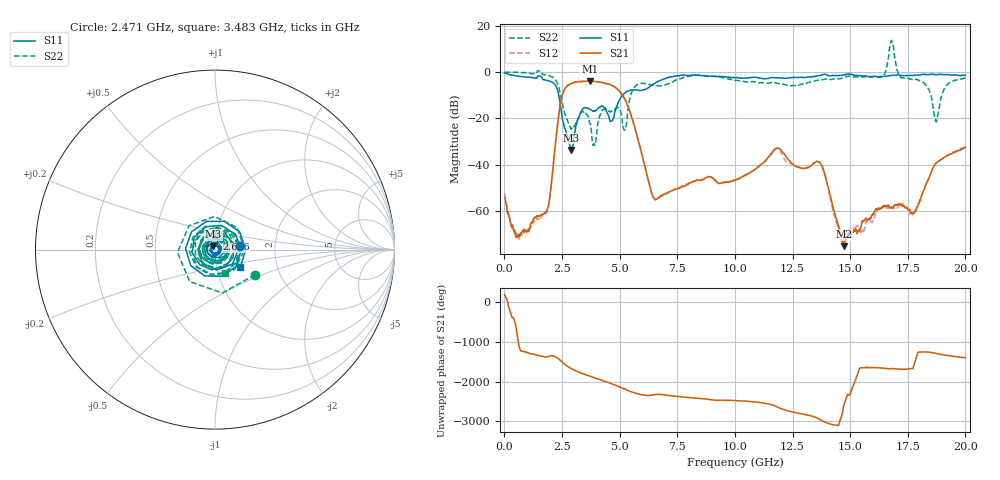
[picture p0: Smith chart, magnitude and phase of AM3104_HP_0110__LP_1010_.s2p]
!Created with skrf (http://scikit-rf.org).
# Hz S RI R 50.0
!freq ReS11 ImS11 ReS21 ImS21 ReS12 ImS12 ReS22 ImS22
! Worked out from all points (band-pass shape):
!   1601 points, 10 MHz to 20 GHz, reference 50 ohm
!   highest |S21| = -3.88 dB at 3.708 GHz (marker M1); lowest = -75.1 dB at 14.73 GHz (marker M2)
!   |S21| within 3 dB of the highest: 2.646 GHz to 4.847 GHz (2.201 GHz wide, 58.7 % of centre)
!   lowest |S11| = -33.6 dB at 2.884 GHz (marker M3), VSWR 1.04, Z = 49.1 + j1.84 ohm
!   |S11| at or under -10 dB: 2.361 GHz to 5.129 GHz (2.768 GHz wide, 73.9 % of centre)
!   |S22| runs from -31.6 to 13.6 dB; largest |S21 - S12| = 0.052
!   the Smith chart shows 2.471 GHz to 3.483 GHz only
!   S11 on the Smith chart (normalised r, x): 2.471 GHz: 1.32, +0.06; 2.646 GHz: 1.02, +0.12; 3.483 GHz: 1.30, -0.26
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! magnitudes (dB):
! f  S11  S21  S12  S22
! 10 MHz  -0.4  -54.1  -52.4  0.0
! 584.7 MHz  -1.7  -71.1  -70.8  -0.1
! 1.809 GHz  -3.5  -60.3  -61.1  -1.2
! 2.471 GHz  -17.1  -11.6  -11.7  -11.6
! 2.646 GHz  -24.6  -6.9  -6.9  -18.6
! 2.884 GHz  -33.6  -5.0  -5.1  -24.5
! 3.346 GHz  -16.7  -4.0  -4.1  -17.3
! 3.483 GHz  -15.3  -4.0  -4.0  -17.0
! 3.708 GHz  -16.0  -3.9  -3.9  -22.0
! 4.658 GHz  -21.0  -5.7  -5.8  -16.8
! 5.17 GHz  -9.5  -10.7  -10.7  -24.4
! 5.682 GHz  -7.6  -24.9  -24.9  -6.0
! 6.682 GHz  -4.0  -54.4  -54.1  -5.9
! 10.01 GHz  -2.5  -46.8  -46.8  -3.6
! 11.82 GHz  -2.5  -32.8  -32.9  -4.8
! 13.34 GHz  -2.1  -40.1  -40.1  -4.1
! 13.8 GHz  -1.1  -41.1  -40.8  -3.3
! 14.73 GHz  -1.2  -75.1  -71.5  -2.4
! 16.68 GHz  -1.6  -57.9  -58.7  7.3
! 17.78 GHz  -1.3  -60.7  -60.1  -3.1
! 18.73 GHz  -1.2  -39.3  -39.4  -21.4
! 20 GHz  -1.4  -32.4  -32.1  -2.6
